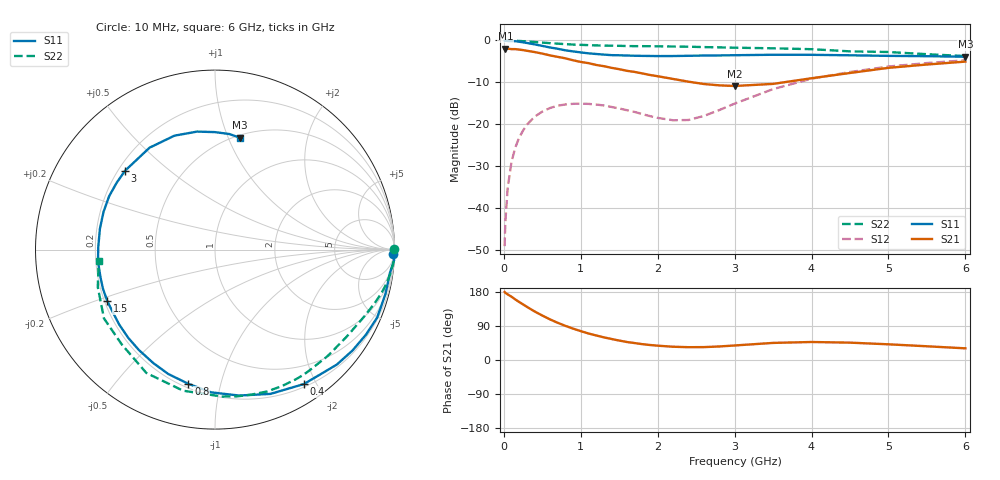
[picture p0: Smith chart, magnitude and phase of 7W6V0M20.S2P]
! Infineon Technologies  Discrete & RF Semiconductors
! BFS17W
! Si NPN RF Bipolar Junction Transistor in SOT323
! VCE = 6 V  IC = 0.2 mA
! Common Emitter S-Parameters:  August  1999
# GHz  S  MA  R  50
!  f  S11  S21  S12  S22
! GHz  MAG  ANG  MAG  ANG  MAG  ANG  MAG  ANG
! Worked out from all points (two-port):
!   36 points, 10 MHz to 6 GHz, reference 50 ohm
!   highest |S21| = -1.94 dB at 20 MHz (marker M1); lowest = -10.9 dB at 3 GHz (marker M2)
!   |S21| within 3 dB of the highest: start of sweep to 951.9 MHz
!   lowest |S11| = -3.9 dB at 6 GHz (marker M3), VSWR 4.53, Z = 26.2 + j55.1 ohm
!   |S11| at or under -10 dB: nowhere
!   |S22| runs from -3.7 to 0.0 dB; largest |S21 - S12| = 0.8
!   S11 on the Smith chart (normalised r, x): 10 MHz: 34, -72; 400 MHz: 0.24, -1.84; 800 MHz: 0.22, -0.80; 1.5 GHz: 0.21, -0.22; 3 GHz: 0.23, +0.36; 6 GHz: 0.52, +1.10
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0.01  0.9895 -1.3  0.796 179.5  0.0035 86.2  0.9999 0.1
0.02  0.9999 -3.3  0.8 177.3  0.0069 90.9  0.9906 -0.6
0.05  0.9834 -7.5  0.799 173.2  0.0174 86.3  0.9982 -1.9
0.1  0.9814 -14.6  0.788 166.9  0.0357 80.7  0.9977 -3.9
0.15  0.9797 -22.7  0.788 159.7  0.053 75.9  0.9915 -5.8
0.25  0.9503 -36.3  0.767 146.7  0.0841 66.8  0.9798 -9.5
0.4  0.8981 -56.5  0.727 128.1  0.123 55.5  0.959 -14.6
0.5  0.8612 -69.0  0.697 117.3  0.1415 48.6  0.9428 -17.6
0.6  0.8242 -80.6  0.663 107.2  0.1561 42.4  0.9282 -20.4
0.8  0.7624 -101.2  0.612 90.1  0.1722 32.5  0.9038 -25.8
1.1  0.702 -127.2  0.536 70.0  0.1749 21.9  0.8794 -33.5
1.5  0.6651 -154.6  0.454 51.3  0.1541 15.4  0.8625 -43.9
1.8  0.6543 -171.7  0.404 41.8  0.1321 17.1  0.8546 -52.4
2.2  0.6517 169.7  0.347 35.0  0.1115 33.0  0.847 -63.7
2.6  0.6606 153.2  0.302 34.0  0.1255 56.8  0.8331 -75.8
3  0.6665 138.7  0.286 38.3  0.1761 68.9  0.8192 -87.4
3.5  0.6748 122.7  0.303 45.1  0.2626 69.9  0.806 -102.7
4  0.6738 109.6  0.354 47.5  0.3494 63.9  0.7866 -119.1
4.5  0.665 98.6  0.409 45.8  0.4199 56.2  0.7409 -134.5
5  0.6545 90.0  0.471 41.4  0.4885 48.6  0.7278 -148.2
5.5  0.6488 82.9  0.516 36.2  0.5376 41.1  0.6854 -162.3
6  0.6386 77.5  0.559 30.8  0.58 34.2  0.6511 -174.5
